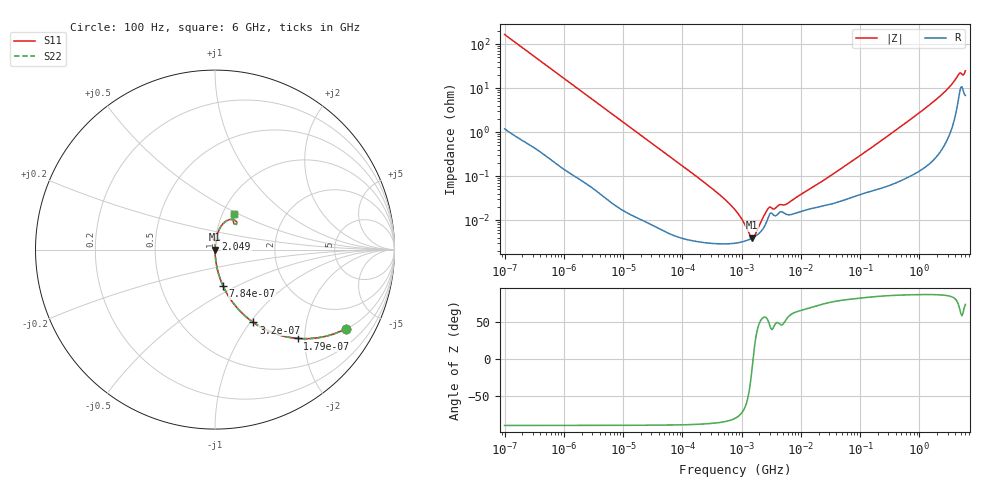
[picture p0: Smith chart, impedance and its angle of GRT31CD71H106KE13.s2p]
!Murata Part Number: GRT31CD71H106KE13
!These Parameters are Measured in Series Mode Connection
!Data Generated on Jun 19, 2026
!  o--ll--o
!Port1  Port2
!  o------o
!Operation Temp=25[degC], DC Bias Voltage=0[V]
!Freq. Start=100[Hz] Stop=6[GHz] 401[Steps]
# Hz S RI R 50
!Freq.(Hz) S11(Real) S11(Imag) S21(Real) S21(Imag) S12(Real) S12(Imag) S22(Real) S22(Imag)
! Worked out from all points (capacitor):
!   401 points, 100 Hz to 6 GHz, reference 50 ohm
!   read as one part in series: C = 9.63 uF near 109 Hz
!   lowest |Z| = 3.96 mohm at 1.516 MHz (marker M1)
!   series resonance near 1.562 MHz, so ESL is about 1.1 nH
!   S11 on the Smith chart (normalised r, x): 100 Hz: 1.02, -3.30; 179 Hz: 1.01, -1.85; 320 Hz: 1.01, -1.04; 784 Hz: 1.00, -0.43; 2.049 GHz: 1.01, +0.12; 6 GHz: 1.14, +0.47
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100  0.7301 -0.4403  0.2699 0.4403  0.2699 0.4403  0.7301 -0.4403
179  0.4612 -0.4947  0.5388 0.4947  0.5388 0.4947  0.4612 -0.4947
320  0.2136 -0.4057  0.7864 0.4057  0.7864 0.4057  0.2136 -0.4057
479  0.1096 -0.3082  0.8904 0.3082  0.8904 0.3082  0.1096 -0.3082
784  0.0449 -0.2028  0.9551 0.2028  0.9551 0.2028  0.0449 -0.2028
2008  0.00768 -0.0828  0.9923 0.0828  0.9923 0.0828  0.00768 -0.0828
40335  8.18e-05 -0.00423  0.9999 0.00423  0.9999 0.00423  8.18e-05 -0.00423
330837  2.96e-05 -0.000498  1 0.000498  1 0.000498  2.96e-05 -0.000498
774597  2.98e-05 -0.000169  1 0.000169  1 0.000169  2.98e-05 -0.000169
1059725  3.24e-05 -8.87e-05  1 8.87e-05  1 8.87e-05  3.24e-05 -8.87e-05
1516199  3.9e-05 -6.7e-06  1 6.7e-06  1 6.7e-06  3.9e-05 -6.7e-06
2074311  5.33e-05 6.7e-05  0.9999 -6.7e-05  0.9999 -6.7e-05  5.33e-05 6.7e-05
2967816  0.000135 0.000142  0.9999 -0.000142  0.9999 -0.000142  0.000135 0.000142
3549919  0.000127 0.000126  0.9999 -0.000126  0.9999 -0.000126  0.000127 0.000126
4440638  0.000152 0.000165  0.9998 -0.000165  0.9998 -0.000165  0.000152 0.000165
5809218  0.000134 0.00019  0.9999 -0.00019  0.9999 -0.00019  0.000134 0.00019
1.555665e7  0.000184 0.000516  0.9998 -0.000516  0.9998 -0.000516  0.000184 0.000516
3.124326e8  0.000684 0.00863  0.9993 -0.00863  0.9993 -0.00863  0.000684 0.00863
2.048624e9  0.0064 0.0584  0.9936 -0.0584  0.9936 -0.0584  0.0064 0.0584
3.505958e9  0.0252 0.1156  0.9748 -0.1156  0.9748 -0.1156  0.0252 0.1156
4.586474e9  0.0839 0.1681  0.9161 -0.1681  0.9161 -0.1681  0.0839 0.1681
6e9  0.1074 0.1982  0.8926 -0.1982  0.8926 -0.1982  0.1074 0.1982
